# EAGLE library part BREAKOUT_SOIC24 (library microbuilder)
Chip Breakout - SOIC24 (Dual-Width)
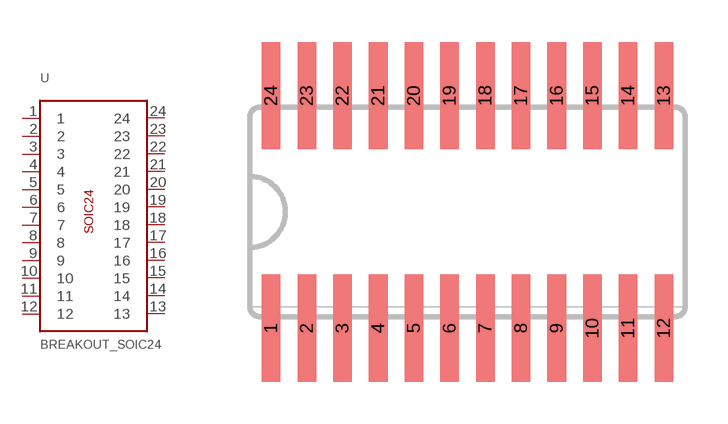
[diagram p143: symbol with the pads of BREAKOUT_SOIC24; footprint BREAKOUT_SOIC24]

Designator prefix U

## BREAKOUT_SOIC24  [BREAKOUT_SOIC24]
1  1
2  2
3  3
4  4
5  5
6  6
7  7
8  8
9  9
10  10
11  11
12  12
13  13
14  14
15  15
16  16
17  17
18  18
19  19
20  20
21  21
22  22
23  23
24  24

## Footprint BREAKOUT_SOIC24 (pad centres in mm)
smd 0.66 x 3.81: 1 -6.985,-4.14; 2 -5.715,-4.14; 3 -4.445,-4.14; 4 -3.175,-4.14; 5 -1.905,-4.14; 6 -0.635,-4.14; 7 0.635,-4.14; 8 1.905,-4.14; 9 3.175,-4.14; 10 4.445,-4.14; 11 5.715,-4.14; 12 6.985,-4.14; 13 6.985,4.14; 14 5.715,4.14; 15 4.445,4.14; 16 3.175,4.14; 17 1.905,4.14; 18 0.635,4.14; 19 -0.635,4.14; 20 -1.905,4.14; 21 -3.175,4.14; 22 -4.445,4.14; 23 -5.715,4.14; 24 -6.985,4.14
